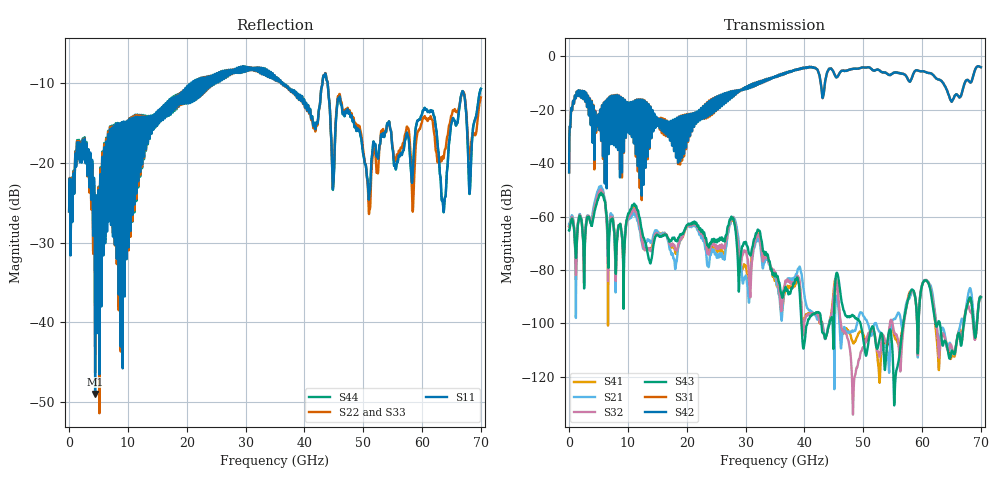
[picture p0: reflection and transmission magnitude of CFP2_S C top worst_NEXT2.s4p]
! AWR Design Environment (8415) Tue Jan 08 13:14:25 2019
! Document = 'CFP2 Channel_S'
! nPorts: 4, nXvals: 7001
# HZ S DB R 50
!Freq DBS11 AngS11 DBS12 AngS12 DBS13 AngS13 DBS14 AngS14
!	DBS21 AngS21 DBS22 AngS22 DBS23 AngS23 DBS24 AngS24
!	DBS31 AngS31 DBS32 AngS32 DBS33 AngS33 DBS34 AngS34
!	DBS41 AngS41 DBS42 AngS42 DBS43 AngS43 DBS44 AngS44
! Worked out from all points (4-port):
!   7000 points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, 10 MHz to 70 GHz, reference 50 ohm
!   strongest paths, dB at 10 MHz, 17.51 GHz, 35.01 GHz, 52.51 GHz, 70 GHz:
!     S42: -43.5, -33.5, -7.5, -5.0, -4.0
!     S31: -43.4, -32.7, -7.5, -5.0, -4.0
!     S43: -65.2, -68.2, -81.9, -108.8, -90.1
!     S32: -63.9, -70.2, -81.2, -110.6, -90.0
!     S21: -62.9, -73.8, -82.8, -102.2, -90.4
!     S41: -63.7, -70.9, -84.0, -114.5, -90.5
!   lowest |S11| = -49.0 dB at 4.43 GHz (marker M1), VSWR 1.01, Z = 49.9 + j0.337 ohm
!   |S11| at or under -10 dB: start of sweep to 20.77 GHz; 36.28 GHz to 43.07 GHz (6.792 GHz wide, 17.1 % of centre); 43.96 GHz to end of sweep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
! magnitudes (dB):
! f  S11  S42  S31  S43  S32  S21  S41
! 10 MHz  -26.1  -43.5  -43.4  -65.2  -63.9  -62.9  -63.7
! 1.32 GHz  -18.0  -13.1  -13.2  -69.5  -69.5  -69.2  -69.8
! 4.43 GHz  -49.0  -20.8  -20.4  -57.3  -55.6  -53.8  -55.3
! 18.01 GHz  -12.5  -23.4  -23.6  -68.7  -72.0  -79.1  -73.1
! 27.89 GHz  -8.3  -14.2  -14.1  -60.6  -60.3  -60.2  -61.1
! 29.65 GHz  -8.4  -12.2  -12.3  -70.0  -73.2  -84.1  -78.4
! 70 GHz  -10.7  -4.0  -4.0  -90.1  -90.0  -90.4  -90.5
